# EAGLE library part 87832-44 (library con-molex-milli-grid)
HEADER
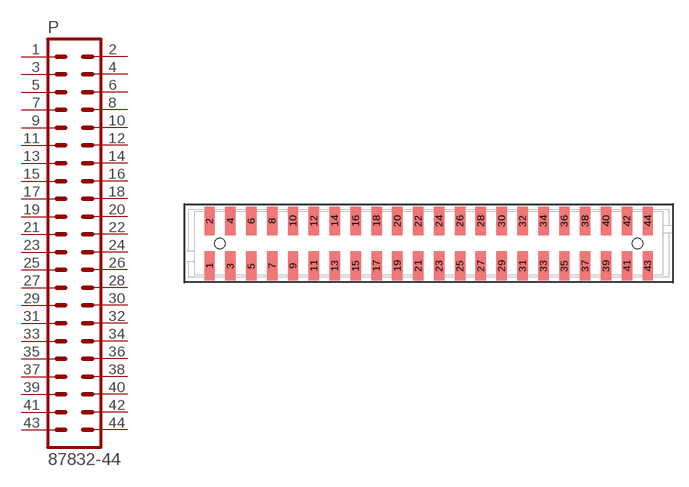
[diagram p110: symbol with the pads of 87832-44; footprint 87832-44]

Designator prefix P

## 87832-44  [87832-44]
1  1  pas
2  2  pas
3  3  pas
4  4  pas
5  5  pas
6  6  pas
7  7  pas
8  8  pas
9  9  pas
10  10  pas
11  11  pas
12  12  pas
13  13  pas
14  14  pas
15  15  pas
16  16  pas
17  17  pas
18  18  pas
19  19  pas
20  20  pas
21  21  pas
22  22  pas
23  23  pas
24  24  pas
25  25  pas
26  26  pas
27  27  pas
28  28  pas
29  29  pas
30  30  pas
31  31  pas
32  32  pas
33  33  pas
34  34  pas
35  35  pas
36  36  pas
37  37  pas
38  38  pas
39  39  pas
40  40  pas
41  41  pas
42  42  pas
43  43  pas
44  44  pas

## Footprint 87832-44 (pad centres in mm)
HEADER SMD Dual Row, Shrouded, Vertical
smd 1 x 2.75: 1 -21,-2.15; 2 -21,2.15; 3 -19,-2.15; 4 -19,2.15; 5 -17,-2.15; 6 -17,2.15; 7 -15,-2.15; 8 -15,2.15; 9 -13,-2.15; 10 -13,2.15; 11 -11,-2.15; 12 -11,2.15; 13 -9,-2.15; 14 -9,2.15; 15 -7,-2.15; 16 -7,2.15; 17 -5,-2.15; 18 -5,2.15; 19 -3,-2.15; 20 -3,2.15; 21 -1,-2.15; 22 -1,2.15; 23 1,-2.15; 24 1,2.15; 25 3,-2.15; 26 3,2.15; 27 5,-2.15; 28 5,2.15; 29 7,-2.15; 30 7,2.15; 31 9,-2.15; 32 9,2.15; 33 11,-2.15; 34 11,2.15; 35 13,-2.15; 36 13,2.15; 37 15,-2.15; 38 15,2.15; 39 17,-2.15; 40 17,2.15; 41 19,-2.15; 42 19,2.15; 43 21,-2.15; 44 21,2.15
hole 1 at -20,0
hole 1 at 20,0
